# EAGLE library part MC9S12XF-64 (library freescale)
MC9S12XF512 Source: www.freescale.com .. MC9S12XF512V1RM.pdf
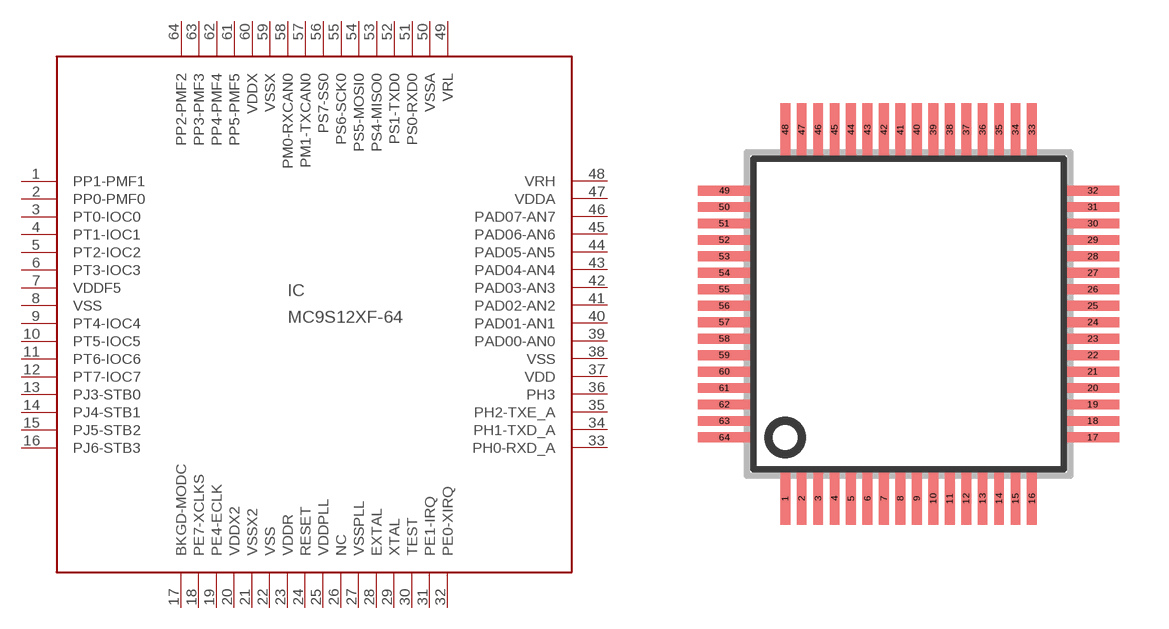
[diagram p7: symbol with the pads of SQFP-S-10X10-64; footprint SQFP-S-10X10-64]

Designator prefix IC

## MC9S12XF-64 (OC_FARNELL: unknown; OC_NEWARK: unknown)  [SQFP-S-10X10-64]
1  PP1-PMF1
2  PP0-PMF0
3  PT0-IOC0
4  PT1-IOC1
5  PT2-IOC2
6  PT3-IOC3
7  VDDF5  pwr
8  VSS  pwr
9  PT4-IOC4
10  PT5-IOC5
11  PT6-IOC6
12  PT7-IOC7
13  PJ3-STB0
14  PJ4-STB1
15  PJ5-STB2
16  PJ6-STB3
17  BKGD-MODC
18  PE7-XCLKS
19  PE4-ECLK
20  VDDX2  pwr
21  VSSX2  pwr
22  VSS  pwr
23  VDDR  pwr
24  RESET
25  VDDPLL  pwr
26  NC  nc
27  VSSPLL  pwr
28  EXTAL  pas
29  XTAL  pas
30  TEST  in
31  PE1-IRQ  in
32  PE0-XIRQ  in
33  PH0-RXD_A
34  PH1-TXD_A
35  PH2-TXE_A
36  PH3
37  VDD  pwr
38  VSS  pwr
39  PAD00-AN0
40  PAD01-AN1
41  PAD02-AN2
42  PAD03-AN3
43  PAD04-AN4
44  PAD05-AN5
45  PAD06-AN6
46  PAD07-AN7
47  VDDA  pwr
48  VRH  pwr
49  VRL  pwr
50  VSSA  pwr
51  PS0-RXD0
52  PS1-TXD0
53  PS4-MISO0
54  PS5-MOSI0
55  PS6-SCK0
56  PS7-SS0
57  PM1-TXCAN0
58  PM0-RXCAN0
59  VSSX  pwr
60  VDDX  pwr
61  PP5-PMF5
62  PP4-PMF4
63  PP3-PMF3
64  PP2-PMF2

## Footprint SQFP-S-10X10-64 (pad centres in mm)
QFP64 shrink quad flat pack, square
smd 0.3 x 1.6: 1 -3.75,-5.6; 2 -3.25,-5.6; 3 -2.75,-5.6; 4 -2.25,-5.6; 5 -1.75,-5.6; 6 -1.25,-5.6; 7 -0.75,-5.6; 8 -0.25,-5.6; 9 0.25,-5.6; 10 0.75,-5.6; 11 1.25,-5.6; 12 1.75,-5.6; 13 2.25,-5.6; 14 2.75,-5.6; 15 3.25,-5.6; 16 3.75,-5.6; 33 3.75,5.6; 34 3.25,5.6; 35 2.75,5.6; 36 2.25,5.6; 37 1.75,5.6; 38 1.25,5.6; 39 0.75,5.6; 40 0.25,5.6; 41 -0.25,5.6; 42 -0.75,5.6; 43 -1.25,5.6; 44 -1.75,5.6; 45 -2.25,5.6; 46 -2.75,5.6; 47 -3.25,5.6; 48 -3.75,5.6
smd 1.6 x 0.3: 17 5.6,-3.75; 18 5.6,-3.25; 19 5.6,-2.75; 20 5.6,-2.25; 21 5.6,-1.75; 22 5.6,-1.25; 23 5.6,-0.75; 24 5.6,-0.25; 25 5.6,0.25; 26 5.6,0.75; 27 5.6,1.25; 28 5.6,1.75; 29 5.6,2.25; 30 5.6,2.75; 31 5.6,3.25; 32 5.6,3.75; 49 -5.6,3.75; 50 -5.6,3.25; 51 -5.6,2.75; 52 -5.6,2.25; 53 -5.6,1.75; 54 -5.6,1.25; 55 -5.6,0.75; 56 -5.6,0.25; 57 -5.6,-0.25; 58 -5.6,-0.75; 59 -5.6,-1.25; 60 -5.6,-1.75; 61 -5.6,-2.25; 62 -5.6,-2.75; 63 -5.6,-3.25; 64 -5.6,-3.75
